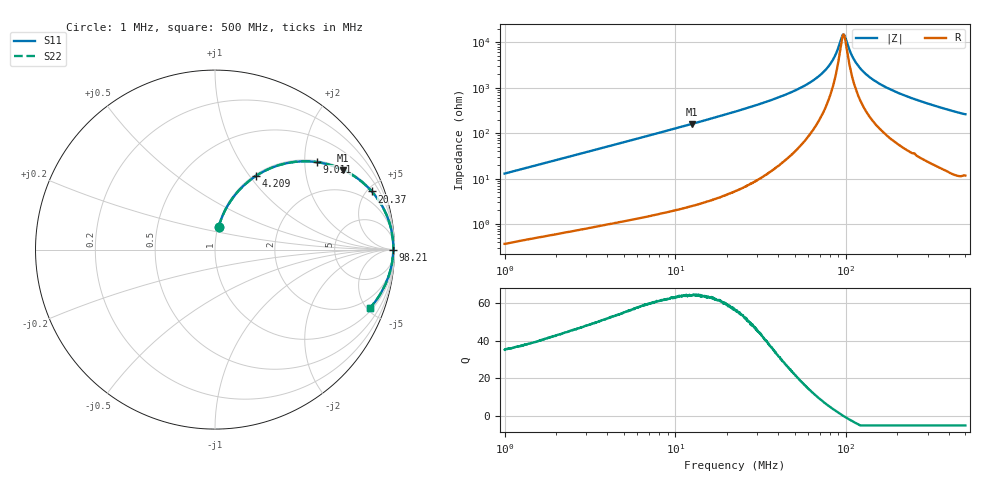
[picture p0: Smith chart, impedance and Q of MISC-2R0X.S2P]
!s-Parameter Generated by FASTRON Sdn. Bhd.
!FASTRON P/N : MISC-2R0X
!Keysight Technologies,E4991B,MY54100416,A.01.15
!Date: Mon Mar 16 10:27:32 2026
!Version  : Rev00 Mon Mar 16 10:27:32 2026
!Data & Calibration Information:
!PortZ  Port1:50+j0  Port2:50+j0
!When reading, reference impedance value at option line is always used.
!Remarks : This data is being provided solely for informational purposes.
!Freq	S11	S21	S12	S22
# Hz S dB R 50
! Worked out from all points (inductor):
!   1601 points, 1 MHz to 500 MHz, reference 50 ohm
!   read as one part in series: L = 2.05 uH near 1.032 MHz
!   highest Q = 64.3 at 12.49 MHz (marker M1), where L = 2.03 uH
!   self-resonance near 96.33 MHz
!   S11 on the Smith chart (normalised r, x): 1 MHz: 1.01, +0.26; 4.209 MHz: 1.02, +1.07; 9.011 MHz: 1.04, +2.29; 20.37 MHz: 1.09, +5.35; 98.21 MHz: open; 500 MHz: 1.23, -5.21
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1000000  -17.86 81.0  -0.10 -7.3  -0.10 -7.3  -17.86 81.0
2820919  -9.47 69.2  -0.59 -19.6  -0.59 -19.6  -9.47 69.2
4208592  -6.60 61.0  -1.16 -27.9  -1.16 -27.9  -6.60 61.0
7957584  -3.04 44.3  -3.12 -44.8  -3.12 -44.8  -3.04 44.3
9010744  -2.53 40.7  -3.71 -48.3  -3.71 -48.3  -2.53 40.7
1.248696e7  -1.50 31.8  -5.56 -57.3  -5.56 -57.3  -1.50 31.8
2.037044e7  -0.62 20.4  -9.17 -68.7  -9.17 -68.7  -0.62 20.4
2.236068e7  -0.51 18.5  -9.96 -70.5  -9.96 -70.5  -0.51 18.5
4.195229e7  -0.15 8.7  -16.41 -79.4  -16.41 -79.4  -0.15 8.7
6.307767e7  -0.07 4.1  -22.90 -81.4  -22.90 -81.4  -0.07 4.1
7.170375e7  -0.06 2.8  -26.10 -80.4  -26.10 -80.4  -0.06 2.8
7.932318e7  -0.06 1.9  -29.66 -77.4  -29.66 -77.4  -0.06 1.9
8.639945e7  -0.06 1.0  -34.29 -69.8  -34.29 -69.8  -0.06 1.0
9.447321e7  -0.06 0.2  -42.41 -29.3  -42.41 -29.3  -0.06 0.2
9.632587e7  -0.06 0.0  -43.45 -5.0  -43.45 -5.0  -0.06 0.0
9.821487e7  -0.06 -0.1  -42.79 20.5  -42.79 20.5  -0.06 -0.1
1.086514e8  -0.06 -1.1  -33.92 68.6  -33.92 68.6  -0.06 -1.1
1.206648e8  -0.07 -2.1  -28.71 76.4  -28.71 76.4  -0.07 -2.1
1.420459e8  -0.09 -3.6  -23.93 79.2  -23.93 79.2  -0.09 -3.6
1.77937e8  -0.12 -5.9  -19.71 79.2  -19.71 79.2  -0.12 -5.9
2.835887e8  -0.28 -11.6  -13.94 75.3  -13.94 75.3  -0.28 -11.6
5e8  -0.72 -20.6  -9.05 66.8  -9.05 66.8  -0.72 -20.6
